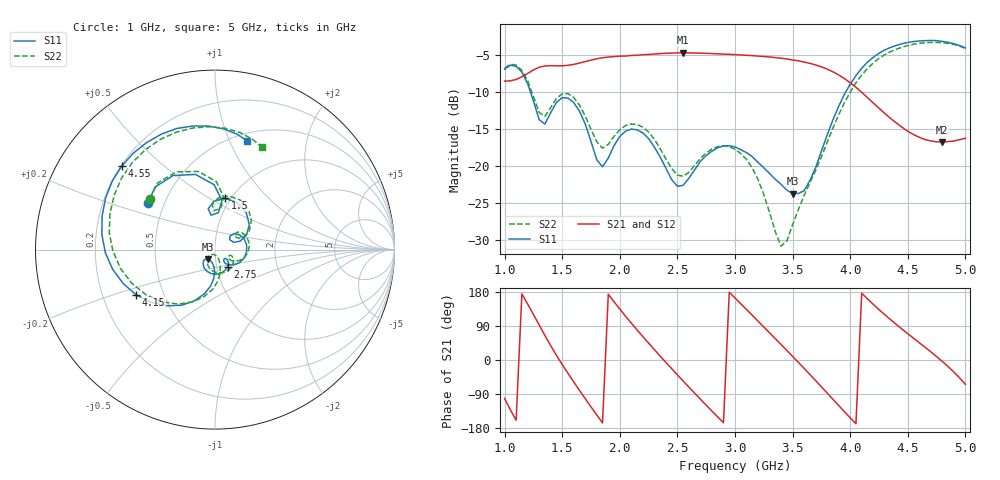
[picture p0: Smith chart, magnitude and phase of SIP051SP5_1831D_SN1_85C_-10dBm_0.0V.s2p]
# GHz  S  dB  R  50
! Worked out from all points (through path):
!   81 points, 1 GHz to 5 GHz, reference 50 ohm
!   highest |S21| = -4.65 dB at 2.55 GHz (marker M1); lowest = -16.7 dB at 4.8 GHz (marker M2)
!   lowest |S11| = -23.7 dB at 3.5 GHz (marker M3), VSWR 1.14, Z = 46 - j4.84 ohm
!   |S11| at or under -10 dB: 1.225 GHz to 3.96 GHz (2.734 GHz wide, 105 % of centre)
!   |S22| runs from -30.8 to -3.2 dB; largest |S21 - S12| = 0.0027
!   S11 on the Smith chart (normalised r, x): 1 GHz: 0.41, +0.27; 1.5 GHz: 0.94, +0.59; 2.75 GHz: 1.13, -0.22; 4.15 GHz: 0.35, -0.24; 4.55 GHz: 0.20, +0.37; 5 GHz: 0.58, +1.17
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1  -6.87 145.2  -8.48 -101.4  -8.47 -101.4  -6.73 142.2
1.15  -7.28 104.5  -7.89 174.5  -7.89 174.7  -7.03 102.1
1.3  -13.70 84.7  -6.61 92.4  -6.61 92.4  -12.72 82.2
1.4  -12.76 99.5  -6.39 37.9  -6.38 37.8  -12.05 93.7
1.5  -10.72 78.7  -6.41 -11.9  -6.39 -12.0  -10.20 75.4
1.7  -14.29 24.7  -5.84 -102.1  -5.83 -102.0  -13.21 29.0
1.9  -18.89 42.1  -5.23 173.6  -5.22 173.6  -17.03 38.6
2.1  -14.97 8.5  -5.01 97.3  -5.00 97.4  -14.29 14.6
2.35  -18.74 -47.8  -4.76 10.5  -4.74 10.6  -17.61 -29.1
2.55  -22.58 -40.9  -4.65 -55.6  -4.63 -55.5  -21.36 -23.1
2.75  -18.55 -53.3  -4.73 -119.2  -4.71 -119.2  -18.22 -32.3
3  -17.39 -99.7  -4.90 163.7  -4.89 163.7  -17.71 -83.1
3.25  -20.21 -132.7  -5.15 87.1  -5.15 87.2  -23.83 -130.0
3.4  -22.45 -134.8  -5.38 40.8  -5.37 40.6  -30.82 -110.3
3.5  -23.70 -126.6  -5.62 9.5  -5.61 9.4  -27.92 -74.1
3.7  -20.19 -92.9  -6.30 -54.3  -6.29 -54.4  -20.57 -72.8
3.95  -10.26 -111.8  -8.14 -136.6  -8.14 -136.5  -11.41 -103.2
4.15  -5.92 -150.0  -10.71 161.3  -10.70 161.3  -6.77 -146.5
4.35  -3.93 172.2  -13.52 106.6  -13.53 106.6  -4.49 170.9
4.55  -3.12 138.2  -15.71 57.4  -15.70 57.5  -3.49 133.4
4.8  -3.10 100.1  -16.73 -3.9  -16.74 -4.1  -3.28 92.6
5  -3.99 73.4  -16.21 -64.2  -16.21 -64.2  -4.04 65.2
